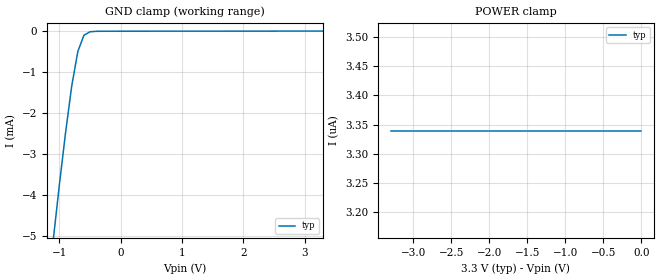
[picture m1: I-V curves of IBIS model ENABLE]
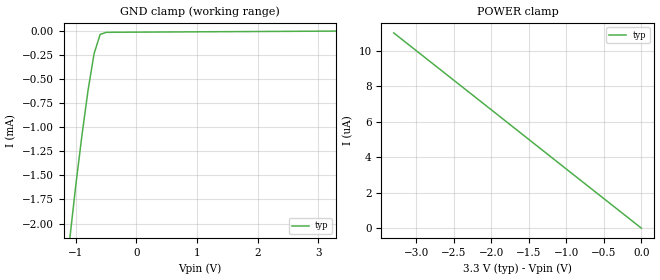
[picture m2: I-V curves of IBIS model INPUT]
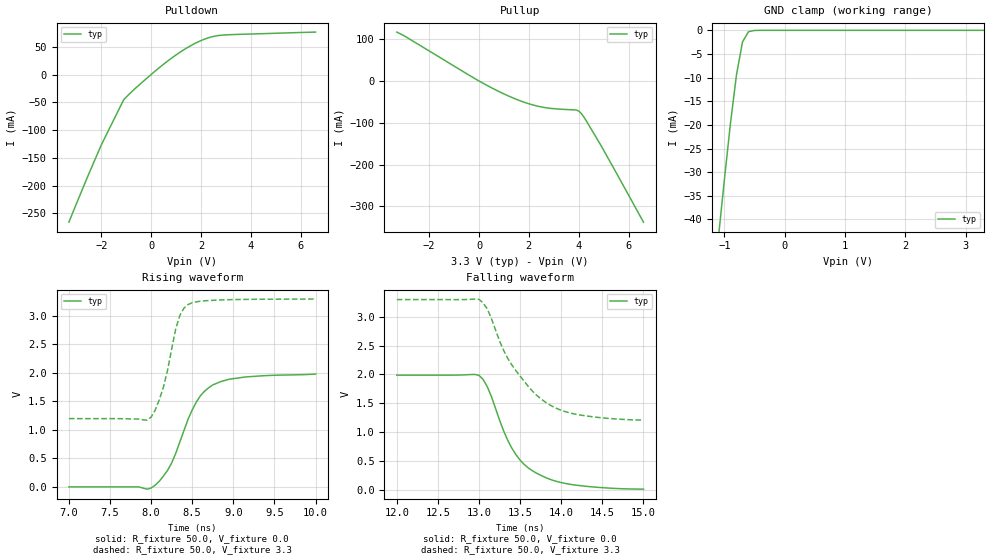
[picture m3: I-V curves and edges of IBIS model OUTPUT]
|   Texas Instruments Incorporated
|   Data Transmissions Products
|   IBIS Model for SN65LVDS388A
|   38DBT TSSOP Package
[IBIS Ver]   3.2
[Comment char]   |_char
[File name]   lvds388a.ibs
[File Rev]   1.0
[Date]   18Oct00
[Source]   File originated at Texas Instruments Incorporated.
   Data Transmission Products Group.
[Notes]
[Disclaimer]
(C) Copyright Texas Instruments Incorporated 2000
   All rights reserved
  Texas Instruments Incorporated hereby grants the user of this IBIS
model a non-exclusive, nontransferable license to use this IBIS model
under the following terms.  Before using this IBIS model, the user
should read this license.  If the user does not accept these terms,
the IBIS model should be returned to Texas Instruments within 30 days.
  The user is granted this license only to use the IBIS model and
is not granted rights to sell, load, rent, lease or license the IBIS
model in whole or in part, or in modified form to anyone other than
user.  User may modify the IBIS model to suit its specific applications
but rights to derivative works and such modifications shall belong to
Texas Instruments.
  This IBIS model is provided on an "AS IS" basis and Texas Instruments
makes absolutely no warranty with respect to the information contained
herein.  TEXAS INSTRUMENTS DISCLAIMS AND CUSTOMER WAIVES ALL WARRANTIES,
EXPRESS OR IMPLIED, INCLUDING WARRANTIES OF MERCHANTABILITY OR FITNESS
FOR A PARTICULAR PURPOSE. The entire risk as to quality and performance
is with the Customer. ACCORDINGLY, IN NO EVENT SHALL THE COMPANY BE LIABLE
FOR ANY DAMAGES, WHETHER IN CONTRACT OR TORT,INCLUDING ANY LOST PROFITS
OR OTHER INCIDENTAL, CONSEQUENTIAL, EXEMPLARY, OR PUNITIVE DAMAGES ARISING
OUT OF THE USE OR APPLICATION OF THE IBIS model provided in this package.
Further, Texas Instruments reserves the right to discontinue or make changes
without notice to any product herein to improve reliability, function, or
design. Texas Instruments does not convey any license under patent rights
or any other intellectual property rights, including those of third parties.
Contact Texas Instruments at ATTN:DATA TRANSMISSIONS
Thomas Fisher 12500 TI Boulevard, M/S 8710  Dallas, Texas 75243
[Copyright]   Copyright 2000, Texas Instruments, All Rights Reserved
[Component]   LVDS388ADBT
[Manufacturer]  Texas Instruments Incorporated
[Package]
|   typ   min   max
R_pkg   0.040   0.035   0.047
L_pkg   2.433nH   1.956nH   3.508nH
C_pkg   0.451pF   0.362pF   0.635pF
[Pin]   signal_name   model_name   R_pin   L_pin   C_pin
1   A1A   INPUT   0.047   3.508n   0.598p
2   A1B   INPUT   0.047   3.231n   0.634p
3   A2A   INPUT   0.046   2.932n   0.570p
4   A2B   INPUT   0.043   2.459n   0.459p
5   AGND   GND   0.035   2.103n   0.387p
6   B1A   INPUT   0.036   2.005n   0.369p
7   B1B   INPUT   0.035   1.956n   0.365p
8   B2A   INPUT   0.036   1.965n   0.364p
9   B2B   INPUT   0.036   1.965n   0.363p
10   AGND   GND   0.036   1.974n   0.362p
11   C1A   INPUT   0.036   1.965n   0.362p
12   C1B   INPUT   0.036   1.965n   0.364p
13   C2A   INPUT   0.036   1.956n   0.365p
14   C2B   INPUT   0.036   2.005n   0.369p
15   AGND   GND   0.035   2.102n   0.387p
16   D1A   INPUT   0.043   2.459n   0.459p
17   D1B   INPUT   0.046   2.932n   0.570p
18   D2A   INPUT   0.047   3.231n   0.634p
19   D2B   INPUT   0.047   3.508n   0.598p
20   GND   GND   0.047   3.508n   0.598p
21   VCC   POWER   0.047   3.231n   0.634p
22   END   ENABLE   0.046   2.932n   0.570p
23   D2Y   OUTPUT   0.043   2.459n   0.458p
24   D1Y   OUTPUT   0.035   2.103n   0.387p
25   ENC   ENABLE   0.036   2.005n   0.369p
26   C2Y   OUTPUT   0.035   1.956n   0.365p
27   C1Y   OUTPUT   0.036   1.965n   0.364p
28   GND   GND   0.036   1.965n   0.363p
29   VCC   POWER   0.036   1.974n   0.363p
30   GND   GND   0.036   1.965n   0.362p
31   B2Y   OUTPUT   0.036   1.965n   0.364p
32   B1Y   OUTPUT   0.036   1.956n   0.365p
33   ENB   ENABLE   0.036   2.004n   0.369p
34   A2Y   OUTPUT   0.035   2.102n   0.387p
35   A1Y   OUTPUT   0.043   2.459n   0.458p
36   ENA   ENABLE   0.046   2.932n   0.570p
37   VCC   POWER   0.047   3.231n   0.635p
38   GND   GND   0.047   3.508n   0.598p
[Diff_pin]   inv_pin   vdiff   tdelay_typ   tdelay_min   tdelay_max
| The 'xxA' pin is Diff_pin and the 'xxB' pin is the inv_pin
1   2   100   0 0 0
3   4   100   0 0 0
6   7   100   0 0 0
8   9   100   0 0 0
11   12   100   0 0 0
13   14   100   0 0 0
16   17   100   0 0 0
18   19   100   0 0 0
| Models and submodels in the file (3): ENABLE (Input), INPUT (Input), OUTPUT (3-state)
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|   Enable Model
[Model]   ENABLE
Model_type   Input
|Signals   ENA,ENB,ENC,END
Vinh = 2.0
Vinl = 0.8
|   typ   min   max
C_comp   1.0pF   NA   NA
|   typ   min   max
[Temperature Range]   25.0   NA   NA
[Voltage range]   3.3V   3.0V   3.6V
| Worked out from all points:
|   GND clamp passes 1 mA (typ) near -0.76 V on its own axis
[GND_clamp]
|   Voltage   I(typ)   I(min)   I(max)
-3.3V     -43.1mA    NA         NA
-1.1V     -5.08mA    NA         NA
-1V       -3.73mA    NA         NA
-900mV    -2.47mA    NA         NA
-800mV    -1.34mA    NA         NA
-700mV    -493uA     NA         NA
-600mV    -98.5uA    NA         NA
-500mV    -13.3uA    NA         NA
3.3V      3.34uA     NA         NA
[Power_clamp]
| Note that the[POWER_clamp]voltage table is referenced to Vcc
| and is calculated using Vtable=Vcc - Vmeasured.
|   Voltage   I(typ)   I(min)   I(max)
-3.3V     3.34uA     NA         NA
-2.7V     3.34uA     NA         NA
-2V       3.34uA     NA         NA
-800mV    3.34uA     NA         NA
0V        3.34uA     NA         NA
|   Receiver Input Model
[Model]   INPUT
Model_type   Input
|Signals   A1A,A1B,A2A,A2B,B1A,B1B,B2A,B2B,
|   C1A,C1B,C2A,C2B,D1A,D1B,D2A,D2B
Vinh = 2.0
Vinl = 0.8
|   typ   min   max
C_comp   1.0pF   NA   NA
|   typ   min   max
[Temperature Range]   25.0   NA   NA
[Voltage range]   3.3V   3.0V   3.6V
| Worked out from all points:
|   GND clamp passes 1 mA (typ) near -0.88 V on its own axis
[GND_clamp]
|   Voltage   I(typ)   I(min)   I(max)
-3.3V     -22.5mA    NA         NA
-1.1V     -2.15mA    NA         NA
-1V       -1.59mA    NA         NA
-900mV    -1.08mA    NA         NA
-800mV    -616uA     NA         NA
-700mV    -234uA     NA         NA
-600mV    -34.5uA    NA         NA
-500mV    -13.2uA    NA         NA
-400mV    -12.3uA    NA         NA
3.3V      8.31pA     NA         NA
[Power_clamp]
| Note that the[POWER_clamp]voltage table is referenced to Vcc
| and is calculated using Vtable=Vcc - Vmeasured.
|   Voltage   I(typ)   I(min)   I(max)
-3.3V     11uA       NA         NA
-3V       10uA       NA         NA
-2V       6.67uA     NA         NA
-1V       3.33uA     NA         NA
0V        8.31pA     NA         NA
|   Receiver Output Model
[Model]   OUTPUT
Model_type   3-state
| Signals   A1Y,A2Y,B1Y,B2Y,C1Y,C2Y,D1Y,D2Y
Vmeas = 1.5V   |Reference voltage for timing measurements
Cref = 8pF   |Timing specification test load capacitance value
Vref = 0   |Timing specification test load voltage; GND
| variable   typ   min   max
C_comp   1.0pF   NA   NA
|   typ   min   max
[Temperature Range]   25.0   NA   NA
[Voltage range]   3.3V   3.0V   3.6V
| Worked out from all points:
|   slope of the pulldown table from 0 to 0.495 V, typ, clamps not added: 26.9 ohm
|   slope of the pullup table from 0 to 0.495 V, typ, clamps not added: 30.7 ohm
|   GND clamp passes 1 mA (typ) near -0.63 V on its own axis
|   rising waveform, R_fixture 50.0, V_fixture 0.0: 20-80 % time 352ps typ, NA min, NA max; typ from 0 V to 1.98 V
|   falling waveform, R_fixture 50.0, V_fixture 0.0: 20-80 % time 420ps typ, NA min, NA max; typ from 1.99 V to 0.006 V
|   rising waveform, R_fixture 50.0, V_fixture 3.3: 20-80 % time 202ps typ, NA min, NA max; typ from 1.2 V to 3.3 V
|   falling waveform, R_fixture 50.0, V_fixture 3.3: 20-80 % time 538ps typ, NA min, NA max; typ from 3.3 V to 1.21 V
[Pulldown]
|   Voltage   I(typ)   I(min)   I(max)
-3.3V     -266mA     NA         NA
-2.5V     -179mA     NA         NA
-2V       -127mA     NA         NA
-1.1V     -45.3mA    NA         NA
-600mV    -23.5mA    NA         NA
600mV     22.1mA     NA         NA
1.2V      41.4mA     NA         NA
1.7V      54.7mA     NA         NA
2.1V      63mA       NA         NA
2.5V      68.7mA     NA         NA
3V        71.5mA     NA         NA
6.6V      76.5mA     NA         NA
[Pullup]
|   Voltage   I(typ)   I(min)   I(max)
| Note that the[Pullup]voltage table is referenced to Vcc
| and is calculated using Vtable=Vcc - Vmeasured.
-3.3V     117mA      NA         NA
-3V       108mA      NA         NA
0V        1.74nA     NA         NA
1.3V      -39mA      NA         NA
1.9V      -52.6mA    NA         NA
2.4V      -61mA      NA         NA
3.9V      -69.6mA    NA         NA
4V        -71.8mA    NA         NA
4.1V      -77.6mA    NA         NA
4.3V      -94.9mA    NA         NA
4.9V      -155mA     NA         NA
6.6V      -338mA     NA         NA
[GND_clamp]
|   Voltage   I(typ)   I(min)   I(max)
| Outputs in High Impedance (off)
-3.3V     -346mA     NA         NA
-1.1V     -43.9mA    NA         NA
-1V       -31.5mA    NA         NA
-900mV    -19.7mA    NA         NA
-800mV    -9.41mA    NA         NA
-700mV    -2.45mA    NA         NA
-600mV    -285uA     NA         NA
-400mV    -1.52uA    NA         NA
3.3V      489pA      NA         NA
[POWER_clamp]
|   Voltage   I(typ)   I(min)   I(max)
| Note that the [POWER_clamp] voltage table is referenced to Vcc
| and is calculated using Vtable = Vcc - Vmeasured.
| Outputs in Tri-state.
-3.3V     0A         NA         NA
0V        0A         NA         NA
[Ramp]
|   typ   min   max
dV/dt_r   1.20V/353ps   NA   NA
dV/dt_f   1.26V/540ps   NA   NA
R_load = 50
[Rising Waveform]
R_fixture = 50.0
V_fixture = 0.0
C_fixture = 0p
L_fixture = 0n
|   V(typ)   V(min)   V(max)
7ns       0V         NA         NA
8ns       -20mV      NA         NA
8.2ns     290mV      NA         NA
8.3ns     590mV      NA         NA
8.5ns     1.35V      NA         NA
8.6ns     1.6V       NA         NA
8.7ns     1.74V      NA         NA
8.85ns    1.85V      NA         NA
9.15ns    1.93V      NA         NA
10ns      1.98V      NA         NA
[Falling Waveform]
R_fixture = 50.0
V_fixture = 0.0
C_fixture = 0p
L_fixture = 0n
|   V(typ)   V(min)   V(max)
12ns      1.986V     NA         NA
13ns      1.982V     NA         NA
13.1ns    1.787V     NA         NA
13.3ns    1.016V     NA         NA
13.4ns    716mV      NA         NA
13.5ns    510mV      NA         NA
13.6ns    374mV      NA         NA
13.85ns   184mV      NA         NA
14.05ns   105mV      NA         NA
15ns      6mV        NA         NA
[Rising Waveform]
R_fixture = 50.0
V_fixture = 3.3
C_fixture = 0p
L_fixture = 0n
|   V(typ)   V(min)   V(max)
7ns       1.199V     NA         NA
7.95ns    1.171V     NA         NA
8ns       1.224V     NA         NA
8.05ns    1.349V     NA         NA
8.15ns    1.753V     NA         NA
8.3ns     2.778V     NA         NA
8.35ns    3.011V     NA         NA
8.45ns    3.201V     NA         NA
8.8ns     3.279V     NA         NA
10ns      3.297V     NA         NA
[Falling Waveform]
R_fixture = 50.0
V_fixture = 3.3
C_fixture = 0p
L_fixture = 0n
|   V(typ)   V(min)   V(max)
12ns      3.299V     NA         NA
13ns      3.303V     NA         NA
13.1ns    3.138V     NA         NA
13.25ns   2.58V      NA         NA
13.35ns   2.276V     NA         NA
13.6ns    1.789V     NA         NA
13.75ns   1.577V     NA         NA
13.95ns   1.404V     NA         NA
14.15ns   1.315V     NA         NA
15ns      1.206V     NA         NA
